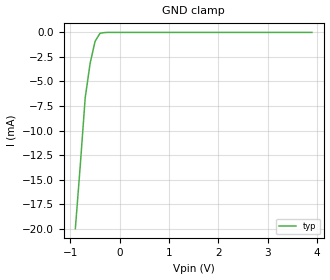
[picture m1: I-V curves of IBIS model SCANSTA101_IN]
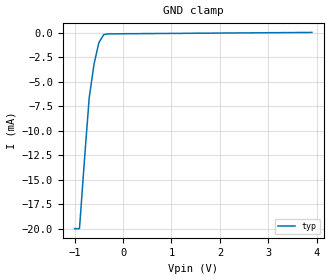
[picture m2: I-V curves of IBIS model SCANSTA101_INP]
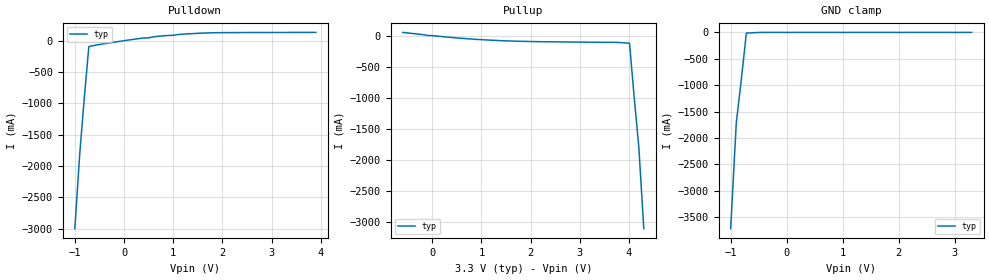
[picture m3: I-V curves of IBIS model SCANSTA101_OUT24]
|   National Semiconductor Corporation
|   System Test Access, Enhanced Solutions
|   IBIS Model of SCANSTA101
|   49 Pin FBGA Package
[IBIS Ver]   2.1
[File name]   sta101sm.ibs
[File Rev]   1.0
[Date]   02/12/02
[Source] File originated at National Semiconductor Corporation
   System Test Access Group/Enhanced Solutions Division
   All data based on simulations,
   except where specified.
[Disclaimer]
(C) Copyright National Semiconductor Corporation 2001
   All rights reserved
National Semiconductor Corporation hereby grants the
user of this IBIS model a non-exclusive, nontransferable
license to use this IBIS model under the following terms.
Before using this IBIS model, the user should read this
license.  If the user does not accept these terms,  the
IBIS model should be returned to National within 30 days.
The user is granted this license only to use the
IBIS model and is not granted rights to sell, load, rent,
lease or license the IBIS model in whole or in part, or in
modified form to anyone other than user. User may modify
the IBIS model to suit its specific applications but rights
to derivative works and such modifications shall belong to
National.
This IBIS model is provided on an "AS IS" basis and
National makes absolutely no warranty with respect to the
information contained herein.NATIONAL DISCLAIMS AND CUSTOMER
WAIVES ALL WARRANTIES, EXPRESS OR IMPLIED, INCLUDING
WARRANTIES OF MERCHANTABILITY OR FITNESS FOR A PARTICULAR
PURPOSE. The entire risk as to quality and performance is
with the Customer. ACCORDINGLY, IN NO EVENT SHALL THE
COMPANY BE LIABLE FOR ANY DAMAGES, WHETHER IN CONTRACT OR
TORT,INCLUDING ANY LOST PROFITS OR OTHER INCIDENTAL,
CONSEQUENTIAL, EXEMPLARY, OR PUNITIVE DAMAGES ARISING OUT
OF THE USE OR APPLICATION OF THE IBIS model provided in
this package.Further, National reserves the right to make
changes without notice to any product herein to improve
reliability, function, or design. National does not convey
any license under patent rights or any other intellectual
property rights, including those of third parties.
National is not obligated to provide maintenance or support
for the licensed IBIS model.
Contact National at ATTN:Enhanced Solutions.
5 Foden Rd, MS 01-50, South Portland, ME 04106
[Copyright]  Copyright 2001, National Semiconductor, All Rights Reserved
[Component]  SCANSTA101
[Manufacturer]  National Semiconductor Corp
[Package]
|   typ   min   max
R_pkg   65.0m   NA   NA
L_pkg   1.50nH   NA   NA
C_pkg   0.08pF   NA   NA
[Pin]   signal_name   model_name   R_pin   L_pin   C_pin
1   CE_B   SCANSTA101_IN
2   RST_B   SCANSTA101_IN
3   TRST_B   SCANSTA101_INP
4   VDD   POWER
5   TDI   SCANSTA101_INP
6   TMS   SCANSTA101_INP
7   A2   SCANSTA101_IN
8   D15   SCANSTA101_IO12
9   OE_B   SCANSTA101_IN
10   TDO   SCANSTA101_OUT24
11   TCK   SCANSTA101_OUT24
12   A0   SCANSTA101_IN
13   A4   SCANSTA101_IN
14   A3   SCANSTA101_IN
15   D13   SCANSTA101_IO12
16   STB_B   SCANSTA101_IN
17   R/W_B   SCANSTA101_IN
18   GND   GND
19   A1   SCANSTA101_IN
20   INT   SCANSTA101_OUT12
21   DTACK_B   SCANSTA101_OUT12
22   GND   GND
23   D14   SCANSTA101_IO12
24   D12   SCANSTA101_IO12
25   NC   NC
26   VDD   POWER
27   TRST0_SM_B   SCANSTA101_OUT24
28   TRIST_SM   SCANSTA101_IO12
29   D11   SCANSTA101_IO12
30   VDD   POWER
31   SCK   SCANSTA101_IN
32   GND   GND
33   TDO_SM   SCANSTA101_OUT24
34   TMS_SM   SCANSTA101_OUT24
35   GND   GND
36   D9   SCANSTA101_IO12
37   D10   SCANSTA101_IO12
38   D7   SCANSTA101_IO12
39   D5   SCANSTA101_IO12
40   D3   SCANSTA101_IO12
41   D1   SCANSTA101_IO12
42   TCK_SM   SCANSTA101_OUT24
43   D8   SCANSTA101_IO12
44   D6   SCANSTA101_IO12
45   D4   SCANSTA101_IO12
46   VDD   POWER
47   D2   SCANSTA101_IO12
48   D0   SCANSTA101_IO12
49   TDI_SM   SCANSTA101_INP
| Models and submodels in the file (5): SCANSTA101_IN (Input), SCANSTA101_INP (Input), SCANSTA101_OUT24 (3-state), SCANSTA101_OUT12 (3-state), SCANSTA101_IO12 (I/O)
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|   Input MODEL
[Model]   SCANSTA101_IN
Model_type   Input
Vinh = 2.0
Vinl = 0.8
|   typ   min   max
C_comp   5.00pF   NA   NA
|   typ   min   max
[Temperature Range]   25.0   NA   NA
[Voltage range]   3.3V   NA   NA
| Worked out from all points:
|   GND clamp passes 1 mA (typ) near -0.50 V on its own axis
[GND_clamp]
| Voltage   I(typ)   I(min)   I(max)
-900mV    -19.99mA   NA         NA
-800mV    -13.52mA   NA         NA
-700mV    -6.65mA    NA         NA
-600mV    -3.14mA    NA         NA
-500mV    -910uA     NA         NA
-400mV    -90uA      NA         NA
-200mV    0A         NA         NA
3.9V      0A         NA         NA
[Power_clamp]
| Voltage   I(typ)   I(min)   I(max)
-3.3V     0A         NA         NA
3.3V      0A         NA         NA
|   Input Pull-up MODEL
[Model]   SCANSTA101_INP
Model_type   Input
Vinh = 2.0
Vinl = 0.8
|   typ   min   max
C_comp   5.00pF   NA   NA
|   typ   min   max
[Temperature Range]   25.0   NA   NA
[Voltage range]   3.3V   NA   NA
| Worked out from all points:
|   GND clamp passes 1 mA (typ) near -0.50 V on its own axis
[GND_clamp]
| Voltage   I(typ)   I(min)   I(max)
-1V       -19.99mA   NA         NA
-900mV    -19.99mA   NA         NA
-800mV    -13.18mA   NA         NA
-700mV    -6.68mA    NA         NA
-600mV    -3.23mA    NA         NA
-500mV    -1.03mA    NA         NA
-400mV    -210uA     NA         NA
-300mV    -130uA     NA         NA
3.9V      20uA       NA         NA
[Power_clamp]
| Voltage   I(typ)   I(min)   I(max)
-3.3V     0A         NA         NA
3.3V      0A         NA         NA
|   3-State Output 24mA MODEL
[Model]   SCANSTA101_OUT24
Model_type   3-state
| Variable   typ   min   max
C_comp   5.00pF   NA   NA
|   typ   min   max
[Temperature Range]   25.0   NA   NA
[Voltage range]   3.3V   NA   NA
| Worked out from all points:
|   slope of the pulldown table from 0 to 0.495 V, typ, clamps not added: 10.9 ohm
|   slope of the pullup table from 0 to 0.495 V, typ, clamps not added: 13.5 ohm
|   GND clamp passes 1 mA (typ) near -0.46 V on its own axis
[Pulldown]
| Voltage   I(typ)   I(min)   I(max)
-1V       -3A        NA         NA
-900mV    -1.8A      NA         NA
-800mV    -844mA     NA         NA
-715mV    -93.6mA    NA         NA
300mV     33mA       NA         NA
1.3V      109.2mA    NA         NA
1.9V      127.5mA    NA         NA
3.9V      132.3mA    NA         NA
[Pullup]
| Voltage   I(typ)   I(min)   I(max)
-600mV    52mA       NA         NA
500mV     -37mA      NA         NA
1.4V      -81mA      NA         NA
3.765V    -108.6mA   NA         NA
4.01V     -122mA     NA         NA
4.1V      -947mA     NA         NA
4.2V      -1.8A      NA         NA
4.3V      -3.1A      NA         NA
[GND_clamp]
| Outputs in Tri-state.
| Voltage   I(typ)   I(min)   I(max)
-1V       -3.72A     NA         NA
-900mV    -1.72A     NA         NA
-800mV    -798mA     NA         NA
-720mV    -13mA      NA         NA
-400mV    -240uA     NA         NA
3.3V      586pA      NA         NA
[POWER_clamp]
| Voltage   I(typ)   I(min)   I(max)
-3.3V     0A         NA         NA
3.3V      0A         NA         NA
[Ramp]
|   typ   min   max
dV/dt_r   1.889/1.12n   NA   NA
dV/dt_f   1.889/0.69n   NA   NA
|[Cload]   30p
R_load = 500ohms
